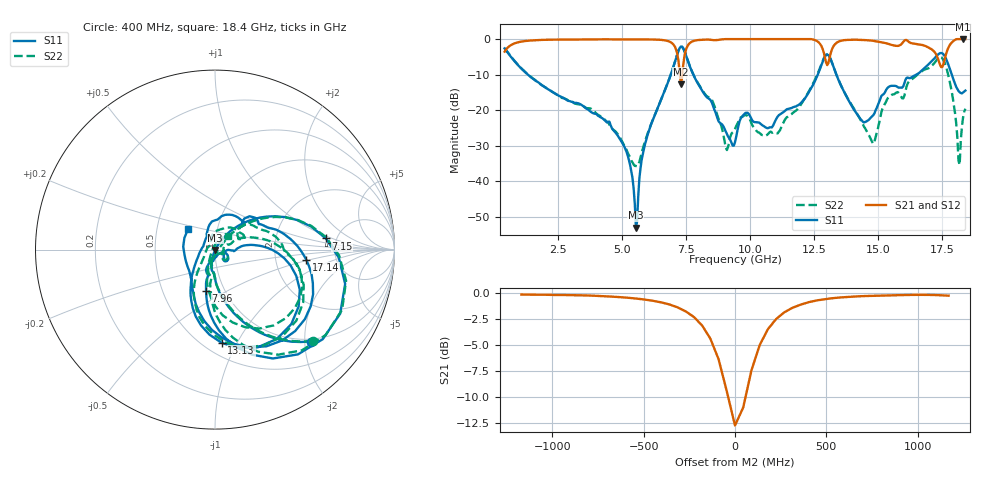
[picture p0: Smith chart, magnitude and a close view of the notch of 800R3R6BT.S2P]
!  American Technical Ceramics  Date:  10/25/10
!  One Norden Lane
!  Huntington Station,  NY.  11746-2102
!  Tel:  (631) 622-4700  Fax:  (631) 622-4748
!  Part Number  800R3R6BT.TXT  Mounting Orientation: Horizontal
!  Description: Ultra Low ESR Microwave Capacitor
!  Application: Coupling, Bypass, Tuning, DC Block, Filters, Matching
# GHZ S DB R 50
! Freq  |S11|  S11 Ph  |S21|  S21 Ph  |S12|  S12 Ph  |S22|  S22 Ph
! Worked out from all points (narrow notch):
!   401 points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, 400 MHz to 18.4 GHz, reference 50 ohm
!   highest |S21| = -0.01 dB at 18.31 GHz (marker M1); lowest = -12.7 dB at 7.285 GHz (marker M2)
!   notch at M2: 12.5 dB deep, 196 MHz wide at half that depth
!   lowest |S11| = -53.0 dB at 5.53 GHz (marker M3), VSWR 1.00, Z = 50.1 - j0.19 ohm
!   |S11| at or under -10 dB: 1.308 GHz to 6.891 GHz (5.583 GHz wide, 136 % of centre); 7.771 GHz to 12.63 GHz (4.862 GHz wide, 47.7 % of centre); 13.36 GHz to 16.48 GHz (3.124 GHz wide, 20.9 % of centre)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
!   |S22| runs from -35.8 to -2.1 dB; largest |S21 - S12| = 0.004
!   S11 on the Smith chart (normalised r, x): 400 MHz: 0.94, -2.13; 7.15 GHz: 4.10, +0.83; 7.96 GHz: 0.82, -0.40; 13.13 GHz: 0.61, -0.87; 17.14 GHz: 3.02, -0.47; 18.4 GHz: 0.72, +0.17
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0.4  -2.63 -43.9  -3.54 46.1  -3.56 46.1  -2.56 -43.0
3.415  -18.57 -98.2  -0.10 -8.6  -0.12 -8.5  -18.66 -95.7
5.035  -29.72 -107.2  -0.07 -19.7  -0.07 -19.6  -29.48 -94.0
5.53  -53.02 -58.1  -0.09 -23.3  -0.09 -23.1  -35.68 -30.5
5.845  -30.82 57.1  -0.08 -25.9  -0.08 -25.8  -29.69 27.4
6.43  -18.47 51.4  -0.18 -32.9  -0.18 -32.8  -18.48 44.3
7.15  -4.14 5.8  -4.35 -63.3  -4.34 -63.2  -4.13 6.5
7.285  -2.12 -27.1  -12.71 -35.6  -12.70 -35.5  -2.12 -25.4
7.96  -12.62 -102.3  -0.28 -17.8  -0.27 -17.6  -12.45 -95.5
9.04  -26.01 -93.2  -0.01 -28.1  -0.01 -27.9  -30.56 -82.8
9.4  -28.98 -31.5  -0.01 -30.2  -0.01 -30.1  -25.29 -25.4
11.065  -21.81 -1.9  -0.01 -45.2  -0.01 -45.2  -26.52 7.7
12.415  -13.31 6.8  -0.07 -63.2  -0.06 -63.2  -12.99 17.6
12.865  -5.64 -25.3  -3.70 -78.8  -3.69 -78.8  -5.48 -21.7
13.135  -5.66 -85.8  -4.08 -31.9  -4.07 -32.0  -5.62 -82.9
14.755  -21.74 126.0  -0.44 -62.0  -0.43 -62.1  -28.90 145.5
15.43  -13.32 63.5  -1.45 -66.3  -1.44 -66.4  -16.09 49.3
17.14  -5.81 -6.4  -3.23 -78.0  -3.21 -78.2  -7.13 -7.2
17.59  -4.77 -70.3  -5.67 -34.2  -5.65 -34.3  -6.66 -68.7
18.13  -14.60 -140.4  -0.01 -49.2  -0.01 -49.4  -34.15 -154.5
18.31  -15.00 174.8  -0.01 -55.6  -0.01 -55.8  -22.00 57.0
18.4  -14.49 142.9  -0.01 -59.2  -0.01 -59.4  -19.58 44.9
